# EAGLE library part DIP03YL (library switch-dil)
DIL/CODE SWITCH
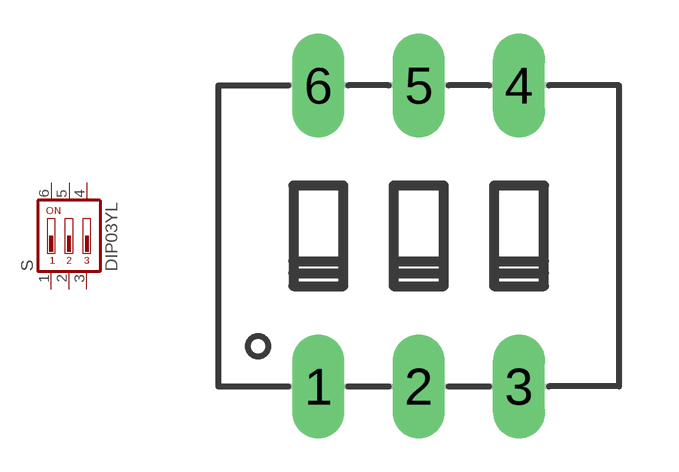
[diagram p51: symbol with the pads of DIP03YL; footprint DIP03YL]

Designator prefix S

## DIP03YL (OC_FARNELL: unknown; OC_NEWARK: unknown)  [DIP03YL]
1  1  pas
2  2  pas
3  3  pas
4  4  pas
5  5  pas
6  6  pas

## Footprint DIP03YL (pad centres in mm)
DIL/CODE SWITCH
drill 0.813 long: 1 -2.54,-3.81; 2 0,-3.81; 3 2.54,-3.81; 4 2.54,3.81; 5 0,3.81; 6 -2.54,3.81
